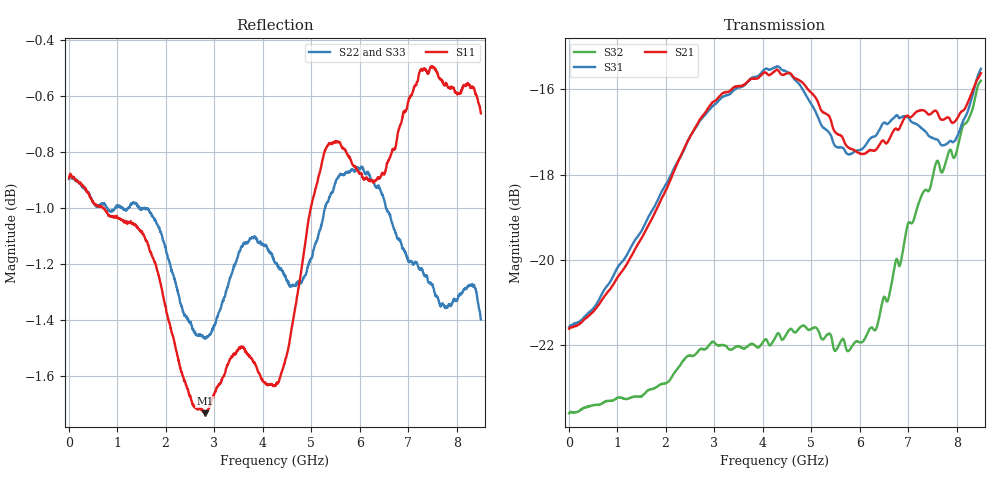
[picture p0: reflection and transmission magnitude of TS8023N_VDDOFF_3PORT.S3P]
!Agilent Technologies,E5071C,MY46522130,B.12.04
!Date: Thu Jul 17 20:35:29 2025
!Data & Calibration Information:
!Freq	S11:SOLT3(ON)	S13:SOLT3(ON)	S14:SOLT3(ON)
!	S31:SOLT3(ON)	S33:SOLT3(ON)	S34:SOLT3(ON)
!	S41:SOLT3(ON)	S43:SOLT3(ON)	S44:SOLT3(ON)
!PortZ  Port1:50+j0  Port3:50+j0  Port4:50+j0
!Above PortZ is port z conversion or system Z0 setting when saving the data.
!When reading, reference impedance value at option line is always used.
# Hz S dB R 50
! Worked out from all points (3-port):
!   1601 points, 10 MHz to 8.5 GHz, reference 50 ohm
!   strongest paths, dB at 10 MHz, 2.132 GHz, 4.255 GHz, 6.378 GHz, 8.5 GHz:
!     S21: -21.6, -18.0, -15.6, -17.4, -15.6
!     S31: -21.6, -18.0, -15.5, -17.0, -15.5
!     S32: -23.6, -22.7, -21.8, -21.5, -15.8
!   lowest |S11| = -1.7 dB at 2.806 GHz (marker M1), VSWR 10.07, Z = 6.43 + j27 ohm
!   |S11| at or under -10 dB: nowhere
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1e7  -0.89 179.8  -21.65 0.0  -21.61 0.1
     -21.62 0.0  -0.90 179.8  -23.60 -0.1
     -21.58 0.1  -23.60 -0.1  -0.91 179.8
1.6231e9  -1.12 156.3  -19.24 6.2  -19.05 4.9
          -19.24 6.2  -1.00 157.3  -23.09 -11.2
          -19.04 4.9  -23.07 -11.5  -1.06 154.8
2.806394e9  -1.73 122.7  -16.56 -7.0  -16.61 -9.0
            -16.56 -7.0  -1.46 134.0  -22.08 -22.7
            -16.60 -9.0  -22.10 -22.9  -1.46 130.8
3.538656e9  -1.50 97.7  -15.93 -21.7  -15.95 -23.0
            -15.93 -21.8  -1.15 116.3  -22.06 -33.5
            -15.95 -23.0  -22.05 -33.9  -1.17 115.2
4.255e9  -1.63 72.0  -15.57 -34.8  -15.46 -37.4
         -15.57 -34.4  -1.19 107.6  -21.80 -38.2
         -15.48 -37.1  -21.83 -38.4  -1.30 103.7
5.252575e9  -0.81 45.3  -16.49 -52.7  -16.85 -55.6
            -16.55 -52.5  -1.03 86.3  -21.86 -49.5
            -16.90 -55.6  -21.87 -49.9  -0.93 82.4
6.441175e9  -0.88 36.5  -17.19 -55.9  -16.84 -59.5
            -17.24 -56.0  -0.94 88.3  -21.03 -47.6
            -16.88 -59.6  -21.13 -47.3  -1.14 82.1
7.168131e9  -0.56 27.6  -16.62 -63.5  -16.88 -70.6
            -16.53 -63.7  -1.20 83.1  -18.74 -55.3
            -16.81 -70.6  -18.86 -55.4  -1.12 69.4
7.868556e9  -0.57 33.4  -16.83 -70.1  -17.24 -73.1
            -16.72 -69.9  -1.35 68.3  -17.64 -67.6
            -17.21 -72.7  -17.42 -66.4  -1.21 64.2
8.5e9  -0.66 41.3  -15.50 -69.1  -15.46 -72.3
       -15.62 -68.7  -1.40 72.5  -15.79 -65.6
       -15.52 -72.3  -15.80 -66.2  -1.51 67.8
